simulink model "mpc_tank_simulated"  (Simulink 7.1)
settings: Solver=ode45  StartTime=0.0  StopTime=400  RelTol=1e-3
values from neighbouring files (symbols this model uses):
  A = [-1/T1 0 A3/(A1*T3) 0    [mpc_controller.m]
  a1 = 0.03    [mpc_controller.m]
  A1 = 4.9    [mpc_controller.m]
  a2 = 0.03    [mpc_controller.m]
  A2 = 4.9    [mpc_controller.m]
  a3 = 0.03    [mpc_controller.m]
  A3 = 4.9    [mpc_controller.m]
  a4 = 0.03    [mpc_controller.m]
  A4 = 4.9    [mpc_controller.m]
  B = [g1*k1/A1 0    [mpc_controller.m]
  g = 981    [mpc_controller.m]
  g1 = 0.3    [mpc_controller.m]
  g2 = 0.3    [mpc_controller.m]
  h1 = 10    [mpc_controller.m]
  h2 = 10    [mpc_controller.m]
  h3 = (k2*v2*(1-g2)/a3)^2/(2*g)    [mpc_controller.m]
  h4 = (k1*v1*(1-g1)/a4)^2/(2*g)    [mpc_controller.m]
  k1 = 1.6    [mpc_controller.m]
  k2 = 1.6    [mpc_controller.m]
  kc = 0.5    [mpc_controller.m]
  md = MPCInit(Ad,Bd,Cyd,Czd,Dzd,Ccd,Dcd,Hp,Hw,zblk,Hu,ublk,  	    du_max,du_min,u_max,u_min,z_max,  	    z_min,Q,R,W,V,Ts,2,'qp_as')    [mpc_controller.m]
  v1 = sqrt(2*g)*((g2-1)*a2*sqrt(h2)+g2*a1*sqrt(h1))/(k1*(g1+g2-1))    [mpc_controller.m]
  v2 = sqrt(2*g)*((g1-1)*a1*sqrt(h1)+g1*a2*sqrt(h2))/(k2*(g1+g2-1))    [mpc_controller.m]
undefined symbols (not defined in the file or in its folder): QuadTank
libraries: simulink x1

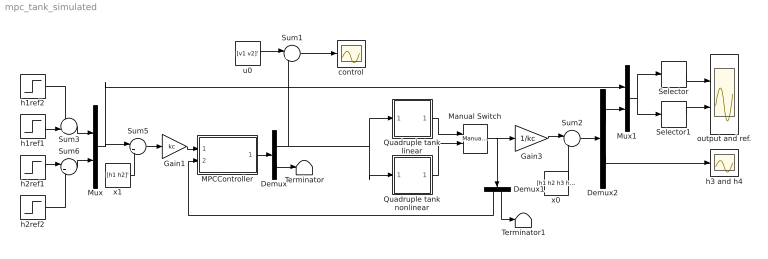
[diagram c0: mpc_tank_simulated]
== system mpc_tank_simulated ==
  Demux : Demux  Outputs=[md.m md.ne]
  Demux1 : Demux  Orientation=down  Outputs=[2 2]
  Demux2 : Demux  Outputs=[2 2]
  Gain1 : Gain  Gain=kc  ParameterDataType=sfix(16)  ParameterScaling=2^0  OutDataType=sfix(16)  OutScaling=2^0
  Gain3 : Gain  Gain=1/kc  ParameterDataType=sfix(16)  ParameterScaling=2^0  OutDataType=sfix(16)  OutScaling=2^0
  MPCController : Subsystem  mask{md=md}
      mask prompts: md "MPCData"
  Manual Switch : simulink/Signal Routing/Manual Switch  SystemSampleTime=-1  sw=0  action=0  varsize=off
  Mux : Mux  Inputs=2
  Mux1 : Mux  Inputs=2
  Quadruple tank linear : Subsystem
  Quadruple tank nonlinear : Subsystem
  Selector : Selector  InputPortWidth=4  IndexOptions=Index vector (dialog)  Indices=[1 3]  OutputSizes=1
  Selector1 : Selector  InputPortWidth=4  IndexOptions=Index vector (dialog)  Indices=[2 4]  OutputSizes=1
  Sum1 : Sum  Inputs=|++  OutDataType=sfix(16)  OutScaling=2^0
  Sum2 : Sum  Inputs=|++  OutDataType=sfix(16)  OutScaling=2^0
  Sum3 : Sum  Inputs=++|  OutDataType=sfix(16)  OutScaling=2^0
  Sum5 : Sum  Inputs=|+-  OutDataType=sfix(16)  OutScaling=2^0
  Sum6 : Sum  Inputs=|++  OutDataType=sfix(16)  OutScaling=2^0
  Terminator : Terminator
  Terminator1 : Terminator
  control : Scope
  h1ref1 : Step  Time=0  After=h1+1
  h1ref2 : Step  Time=120  After=3
  h2ref1 : Step  Time=0  After=h2+3
  h2ref2 : Step  Time=220  ZeroCross=off
  h3 and h4 : Scope
  output and ref. : Scope  NumInputPorts=2
  u0 : Constant  Value=[v1 v2]'  OutDataType=sfix(16)  OutScaling=2^0
  x0 : Constant  Value=[h1 h2 h3 h4]'  OutDataType=sfix(16)  OutScaling=2^0
  x1 : Constant  Value=[h1 h2]'  OutDataType=sfix(16)  OutScaling=2^0
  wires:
  MPCController/1(u) -> Demux/1
  Demux/1 -> Sum1/2, Quadruple tank nonlinear/1(u), Quadruple tank linear/1(u)
  Demux/2 -> Terminator/1
  x1/1 -> Sum5/2
  Mux/1 -> Sum5/1, Mux1/1
  Sum5/1 -> Gain1/1
  Gain1/1 -> MPCController/1(Reference)
  u0/1 -> Sum1/1
  Sum1/1 -> control/1
  Gain3/1 -> Sum2/1
  x0/1 -> Sum2/2
  Manual Switch/1 -> Gain3/1, Demux1/1
  Quadruple tank linear/1(y) -> Manual Switch/1
  Quadruple tank nonlinear/1(y) -> Manual Switch/2
  h1ref1/1 -> Sum3/2
  h2ref1/1 -> Sum6/1
  h2ref2/1 -> Sum6/2
  Sum3/1 -> Mux/1
  Sum6/1 -> Mux/2
  h1ref2/1 -> Sum3/1
  Demux1/2 -> Terminator1/1
  Sum2/1 -> Demux2/1
  Demux2/2 -> h3 and h4/1
  Demux2/1 -> Mux1/2
  Mux1/1 -> Selector/1, Selector1/1
  Selector/1 -> output and ref./1
  Selector1/1 -> output and ref./2
  Demux1/1 -> MPCController/2(Measurements)

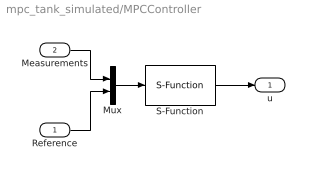
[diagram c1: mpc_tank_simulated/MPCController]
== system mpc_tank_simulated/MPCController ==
  Reference : Inport  OutDataType=sfix(16)  OutScaling=2^0
  Measurements : Inport  Port=2  OutDataType=sfix(16)  OutScaling=2^0
  Mux : Mux  Inputs=2
  S-Function : S-Function  FunctionName=MPCController  Parameters=md  EnableBusSupport=off
  u : Outport  OutDataType=sfix(16)  OutScaling=2^0
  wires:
  S-Function/1 -> u/1
  Reference/1 -> Mux/2
  Measurements/1 -> Mux/1
  Mux/1 -> S-Function/1

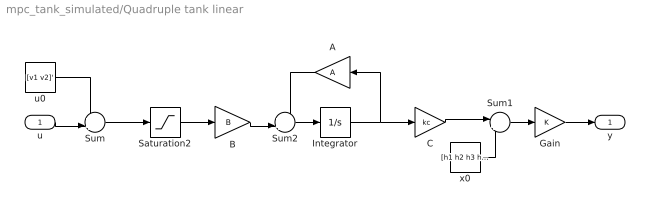
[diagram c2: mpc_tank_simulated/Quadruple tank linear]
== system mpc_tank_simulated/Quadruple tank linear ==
  u : Inport  OutDataType=sfix(16)  OutScaling=2^0
  A : Gain  Orientation=left  Gain=A  Multiplication=Matrix(K*u)  ParameterDataType=sfix(16)  ParameterScaling=2^0  OutDataType=sfix(16)  OutScaling=2^0
  B : Gain  Gain=B  Multiplication=Matrix(K*u)  ParameterDataType=sfix(16)  ParameterScaling=2^0  OutDataType=sfix(16)  OutScaling=2^0
  C : Gain  Gain=kc  ParameterDataType=sfix(16)  ParameterScaling=2^0  OutDataType=sfix(16)  OutScaling=2^0
  Gain : Gain  ParameterDataType=sfix(16)  ParameterScaling=2^0  OutDataType=sfix(16)  OutScaling=2^0
  Integrator : Integrator  InitialCondition=[h1 h2 h3 h4]/kc
  Saturation2 : Saturate  UpperLimit=10  LowerLimit=0
  Sum : Sum  Inputs=++|  OutDataType=sfix(16)  OutScaling=2^0
  Sum1 : Sum  Inputs=|+-  OutDataType=sfix(16)  OutScaling=2^0
  Sum2 : Sum  Inputs=++|  OutDataType=sfix(16)  OutScaling=2^0
  u0 : Constant  Value=[v1 v2]'  OutDataType=sfix(16)  OutScaling=2^0
  x0 : Constant  Value=[h1 h2 h3 h4]'  OutDataType=sfix(16)  OutScaling=2^0
  y : Outport  OutDataType=sfix(16)  OutScaling=2^0
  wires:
  Sum1/1 -> Gain/1
  u/1 -> Sum/2
  u0/1 -> Sum/1
  Sum/1 -> Saturation2/1
  Gain/1 -> y/1
  Saturation2/1 -> B/1
  Integrator/1 -> C/1, A/1
  Sum2/1 -> Integrator/1
  B/1 -> Sum2/2
  C/1 -> Sum1/1
  x0/1 -> Sum1/2
  A/1 -> Sum2/1

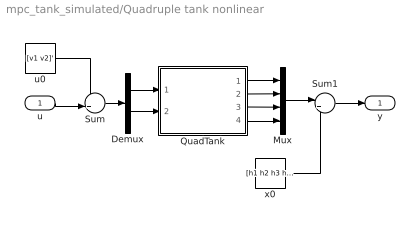
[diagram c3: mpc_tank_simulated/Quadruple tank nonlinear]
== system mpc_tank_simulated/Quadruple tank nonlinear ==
  u : Inport  OutDataType=sfix(16)  OutScaling=2^0
  Demux : Demux  Outputs=2
  Mux : Mux
  QuadTank : Subsystem  AncestorBlock=QuadTank/QuadTank  mask{h0=[h1 h2 h3 h4]', g1=g1, g2=g2, k1=k1, k2=k2}
      mask prompts: h0 "Initial levels"; g1 "Valve 1"; g2 "Valve 2"; k1 "Pump coefficient 1"; k2 "Pump coefficient 2"
  Sum : Sum  Inputs=++|  OutDataType=sfix(16)  OutScaling=2^0
  Sum1 : Sum  Inputs=|+-  OutDataType=sfix(16)  OutScaling=2^0
  u0 : Constant  Value=[v1 v2]'  OutDataType=sfix(16)  OutScaling=2^0
  x0 : Constant  Value=[h1 h2 h3 h4]*kc'  OutDataType=sfix(16)  OutScaling=2^0
  y : Outport  OutDataType=sfix(16)  OutScaling=2^0
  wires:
  QuadTank/4(y4) -> Mux/4
  QuadTank/3(y3) -> Mux/3
  Demux/1 -> QuadTank/1(u1)
  Demux/2 -> QuadTank/2(u2)
  QuadTank/1(y1) -> Mux/1
  QuadTank/2(y2) -> Mux/2
  Sum/1 -> Demux/1
  u0/1 -> Sum/1
  u/1 -> Sum/2
  x0/1 -> Sum1/2
  Sum1/1 -> y/1
  Mux/1 -> Sum1/1

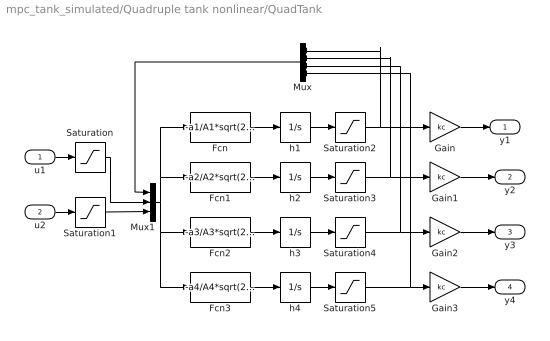
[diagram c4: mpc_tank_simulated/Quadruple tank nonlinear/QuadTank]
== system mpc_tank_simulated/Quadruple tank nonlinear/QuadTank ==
  u1 : Inport  OutDataType=sfix(16)  OutScaling=2^0
  u2 : Inport  Port=2  OutDataType=sfix(16)  OutScaling=2^0
  Fcn : Fcn  Expr=-a1/A1*sqrt(2*g*u[1])+a3/A1*sqrt(2*g*u[3])+g1*k1/A1*u[5]
  Fcn1 : Fcn  Expr=-a2/A2*sqrt(2*g*u[2])+a4/A2*sqrt(2*g*u[4])+g2*k2/A2*u[6]
  Fcn2 : Fcn  Expr=-a3/A3*sqrt(2*g*u[3])+(1-g2)*k2/A3*u[6]
  Fcn3 : Fcn  Expr=-a4/A4*sqrt(2*g*u[4])+(1-g1)*k1/A4*u[5]
  Gain{,1..3} (4 alike) : Gain  Gain=kc  ParameterDataType=sfix(16)  ParameterScaling=2^0  OutDataType=sfix(16)  OutScaling=2^0
  Mux : Mux
  Mux1 : Mux  Inputs=3
  Saturation : Saturate  UpperLimit=10  LowerLimit=0
  Saturation1 : Saturate  UpperLimit=10  LowerLimit=0
  Saturation{2..5} (4 alike) : Saturate  UpperLimit=50  LowerLimit=0
  h1 : Integrator  InitialCondition=h0(1)
  h2 : Integrator  InitialCondition=h0(2)
  h3 : Integrator  InitialCondition=h0(3)
  h4 : Integrator  InitialCondition=h0(4)
  y1 : Outport  OutDataType=sfix(16)  OutScaling=2^0
  y2 : Outport  Port=2  OutDataType=sfix(16)  OutScaling=2^0
  y3 : Outport  Port=3  OutDataType=sfix(16)  OutScaling=2^0
  y4 : Outport  Port=4  OutDataType=sfix(16)  OutScaling=2^0
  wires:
  Saturation5/1 -> Gain3/1, Mux/4
  Saturation4/1 -> Gain2/1, Mux/3
  Saturation3/1 -> Gain1/1, Mux/2
  Saturation2/1 -> Gain/1, Mux/1
  Saturation1/1 -> Mux1/3
  Saturation/1 -> Mux1/2
  Gain/1 -> y1/1
  Gain1/1 -> y2/1
  Gain2/1 -> y3/1
  Gain3/1 -> y4/1
  h4/1 -> Saturation5/1
  h3/1 -> Saturation4/1
  h1/1 -> Saturation2/1
  h2/1 -> Saturation3/1
  Mux/1 -> Mux1/1
  u1/1 -> Saturation/1
  u2/1 -> Saturation1/1
  Fcn/1 -> h1/1
  Fcn1/1 -> h2/1
  Fcn2/1 -> h3/1
  Fcn3/1 -> h4/1
  Mux1/1 -> Fcn/1, Fcn1/1, Fcn2/1, Fcn3/1
